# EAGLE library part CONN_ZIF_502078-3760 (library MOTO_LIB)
CONN ZIF,37CONT,.25MM,1MM HEIGHT,BOTTOM CONT
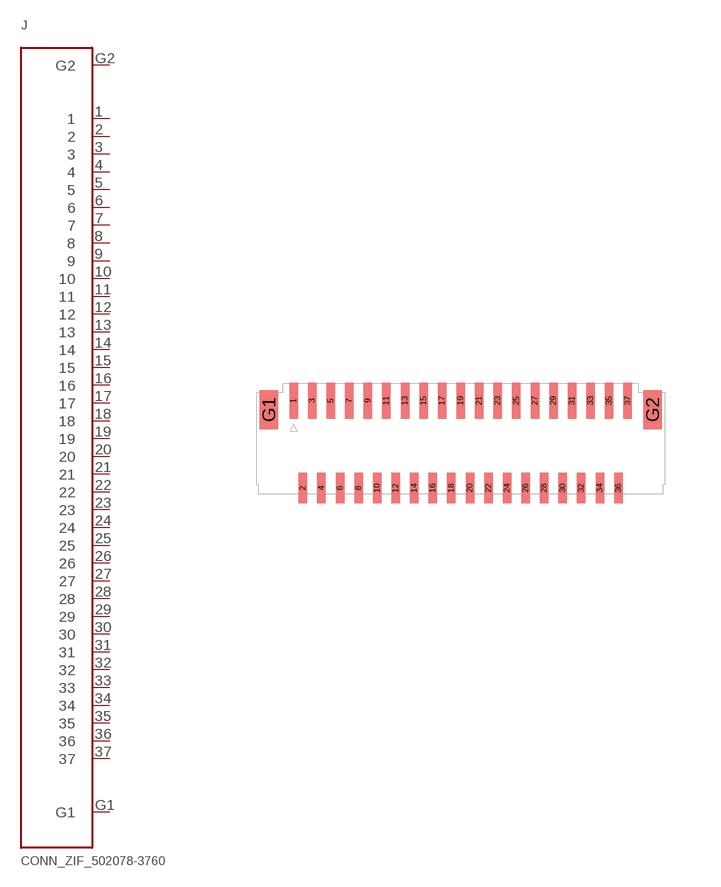
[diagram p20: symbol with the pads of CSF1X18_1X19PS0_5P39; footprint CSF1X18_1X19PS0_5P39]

Designator prefix J

## CONN_ZIF_502078-3760 (MPN: 502078-3760; SUPPLIER: MOLEX)  [CSF1X18_1X19PS0_5P39]
1  1
2  2
3  3
4  4
5  5
6  6
7  7
8  8
9  9
10  10
11  11
12  12
13  13
14  14
15  15
16  16
17  17
18  18
19  19
20  20
21  21
22  22
23  23
24  24
25  25
26  26
27  27
28  28
29  29
30  30
31  31
32  32
33  33
34  34
35  35
36  36
37  37
G1  G1
G2  G2

## Footprint CSF1X18_1X19PS0_5P39 (pad centres in mm)
smd 0.23 x 0.97: 1 -4.5,1.025; 3 -4,1.025; 5 -3.5,1.025; 7 -3,1.025; 9 -2.5,1.025; 11 -2,1.025; 13 -1.5,1.025; 15 -1,1.025; 17 -0.5,1.025; 19 0,1.025; 21 0.5,1.025; 23 1,1.025; 25 1.5,1.025; 27 2,1.025; 29 2.5,1.025; 31 3,1.025; 33 3.5,1.025; 35 4,1.025; 37 4.5,1.025
smd 0.23 x 0.82: 2 -4.25,-1.33; 4 -3.75,-1.33; 6 -3.25,-1.33; 8 -2.75,-1.33; 10 -2.25,-1.33; 12 -1.75,-1.33; 14 -1.25,-1.33; 16 -0.75,-1.33; 18 -0.25,-1.33; 20 0.25,-1.33; 22 0.75,-1.33; 24 1.25,-1.33; 26 1.75,-1.33; 28 2.25,-1.33; 30 2.75,-1.33; 32 3.25,-1.33; 34 3.75,-1.33; 36 4.25,-1.33
smd 0.5 x 1.05: G1 -5.17,0.785; G2 5.17,0.785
